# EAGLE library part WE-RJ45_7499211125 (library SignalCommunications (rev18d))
WE-RJ45 LAN Transformer Characteristics RJ45 Connector with integrated transformer/ common mode choke Available in SMD, THT and THT with USB 350µH min. OCL with 8mA bias Complies with IEEE 802.3 Extended temperature range -40°C to +85°C available PoE/ PoE+ Applications xDSL Modems Embedded PC LAN Applications Hub, Router, Switches Details see: http://katalog.we-online.de/en/pbs/WE-LAN-RJ45/7499211125 Updated by Yingchun Shan 2016-08-30 2016(C) Würth Elektronik
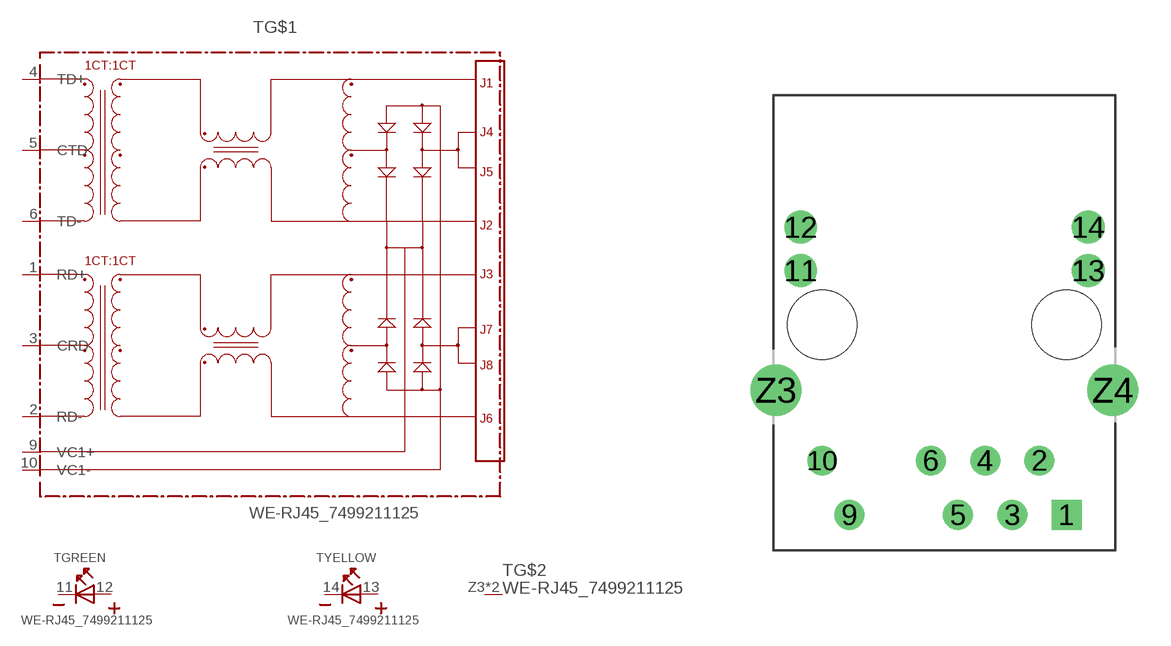
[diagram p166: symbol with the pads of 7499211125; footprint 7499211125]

Designator prefix T; gates G$1=7499211125 G$2=GND_PIN GREEN=LED-2PIN YELLOW=LED-2PIN

## WE-RJ45_7499211125  [7499211125]
1  G$1:RD+
2  G$1:RD-
3  G$1:CRD
4  G$1:TD+
5  G$1:CTD
6  G$1:TD-
9  G$1:VC1+
10  G$1:VC1-
11  GREEN:K  pas
12  GREEN:A  pas
13  YELLOW:A  pas
14  YELLOW:K  pas
Z3  G$2:1  pwr
Z4  G$2:1  pwr

## Footprint 7499211125 (pad centres in mm)
drill 0.89 square: 1 5.715,-8.89
drill 0.89: 2 4.445,-6.35; 3 3.175,-8.89; 4 1.905,-6.35; 5 0.635,-8.89; 6 -0.635,-6.35; 9 -4.445,-8.89; 10 -5.715,-6.35
drill 1.02: 11 -6.725,2.54; 12 -6.725,4.57; 13 6.725,2.54; 14 6.725,4.57
drill 1.6: Z3 -7.875,-3.05; Z4 7.875,-3.05
hole 3.25 at 5.715,0
hole 3.25 at -5.715,0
